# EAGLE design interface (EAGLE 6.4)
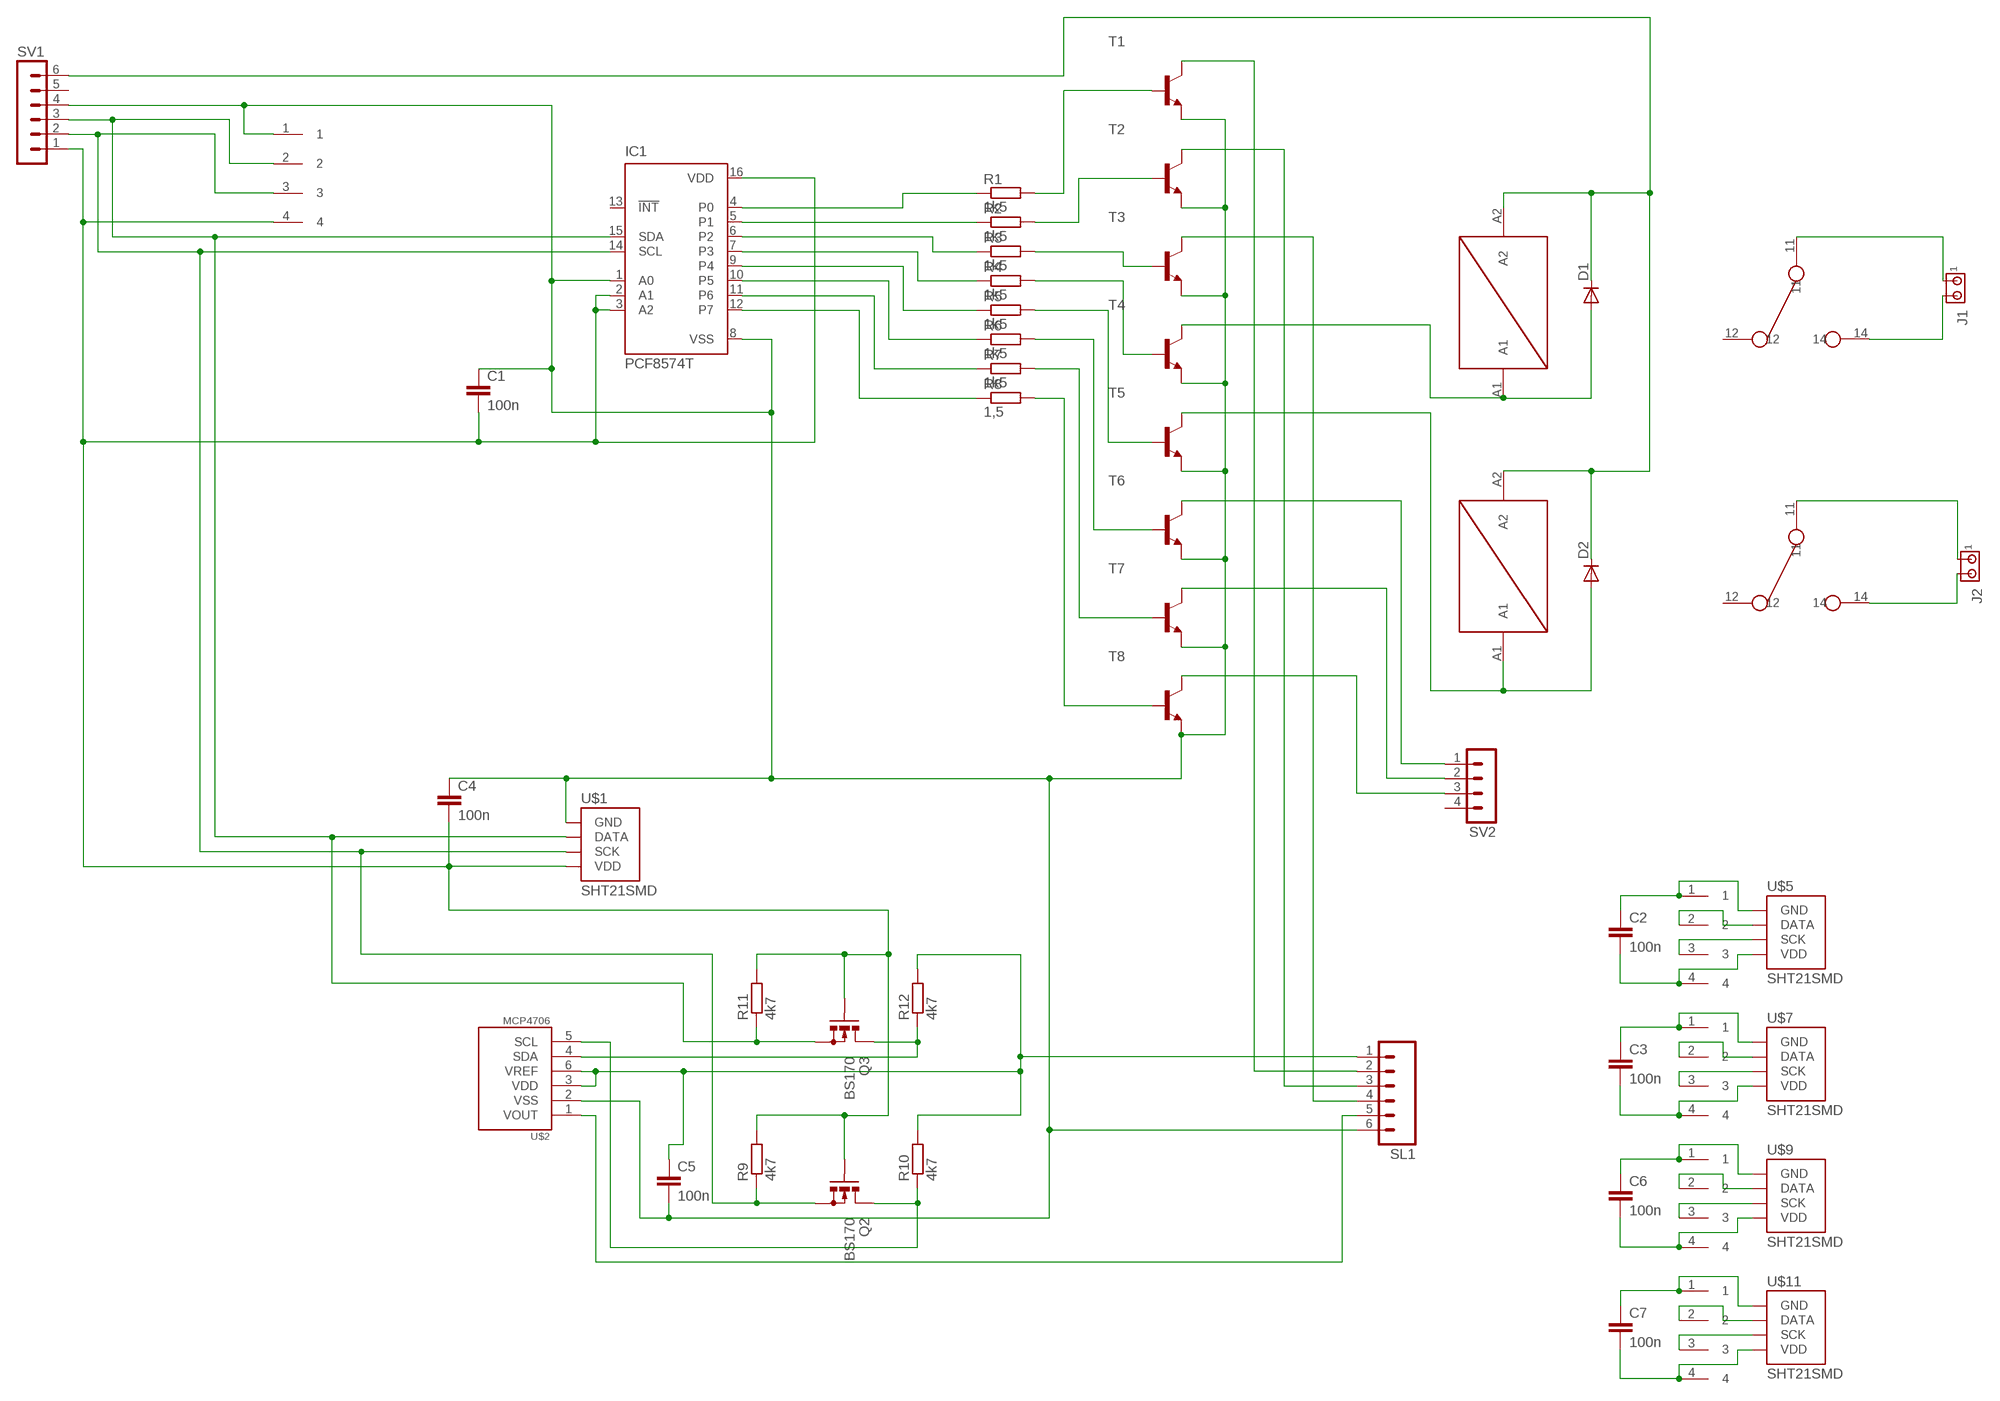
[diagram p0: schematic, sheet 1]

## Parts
C1  100n  C-EUC0805K  [C0805K]
C2  100n  C-EUC0805K  [C0805K]
C3  100n  C-EUC0805K  [C0805K]
C4  100n  C-EUC0805K  [C0805K]
C5  100n  C-EUC0805K  [C0805K]
C6  100n  C-EUC0805K  [C0805K]
C7  100n  C-EUC0805K  [C0805K]
D1  DIODE-MINIMELF  [MINIMELF]
D2  DIODE-MINIMELF  [MINIMELF]
IC1  PCF8574T  [SO16W]
J1  MTA02-156  [1X2MTA]
J2  MTA02-156  [1X2MTA]
Q2  BS170  [SOT54E]
Q3  BS170  [SOT54E]
R1  1k5  R-EU_M0805  [M0805]
R2  1k5  R-EU_M0805  [M0805]
R3  1k5  R-EU_M0805  [M0805]
R4  1k5  R-EU_M0805  [M0805]
R5  1k5  R-EU_M0805  [M0805]
R6  1k5  R-EU_M0805  [M0805]
R7  1k5  R-EU_M0805  [M0805]
R8  1,5  R-EU_M0805  [M0805]
R9  4k7  R-EU_M0805  [M0805]
R10  4k7  R-EU_M0805  [M0805]
R11  4k7  R-EU_M0805  [M0805]
R12  4k7  R-EU_M0805  [M0805]
SL1  MA06  [06PA]
SV1  MA06-1  [MA06-1]
SV2  MA04-1  [MA04-1]
T1  BCW60-NPN-SOT23-BEC  [SOT23-BEC]
T2  BCW60-NPN-SOT23-BEC  [SOT23-BEC]
T3  BCW60-NPN-SOT23-BEC  [SOT23-BEC]
T4  BCW60-NPN-SOT23-BEC  [SOT23-BEC]
T5  BCW60-NPN-SOT23-BEC  [SOT23-BEC]
T6  BCW60-NPN-SOT23-BEC  [SOT23-BEC]
T7  BCW60-NPN-SOT23-BEC  [SOT23-BEC]
T8  BCW60-NPN-SOT23-BEC  [SOT23-BEC]
U$1  SHT21SMD  [SHT21]
U$2  MCP4706  [SOT23-6]
U$3  FINDER_RELAIS  [FINDER_RELAIS]
U$4  FINDER_RELAIS  [FINDER_RELAIS]
U$5  SHT21SMD  [SHT21]
U$6  CON4PIN  [CON4PIN]
U$7  SHT21SMD  [SHT21]
U$8  CON4PIN  [CON4PIN]
U$9  SHT21SMD  [SHT21]
U$10  CON4PIN  [CON4PIN]
U$11  SHT21SMD  [SHT21]
U$12  CON4PIN  [CON4PIN]
U$13  CON4PIN  [CON4PIN]

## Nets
02: SL1.3 T2.C
03: SL1.4 T3.C
5V_ALIX: D1.C D2.C SV1.6 U$3.A2 U$4.A2
5V_LED: C5.1 R10.2 R12.2 SL1.1 U$2.3(VDD) U$2.6(VREF)
GND: C1.1 C4.1 C5.2 IC1.1(A0) IC1.8(VSS) SL1.6 SV1.4 T1.E T2.E T3.E T4.E T5.E T6.E T7.E T8.E U$1.5(GND) U$2.2(VSS) U$13.1
GND_CON: C2.1 U$5.5(GND) U$6.1
GND_CON1: C3.1 U$7.5(GND) U$8.1
GND_CON2: C6.1 U$9.5(GND) U$10.1
GND_CON3: C7.1 U$11.5(GND) U$12.1
N$1: D1.A T4.C U$3.A1
N$2: SV2.1 T6.C
N$3: IC1.4(P0) R1.1
N$4: IC1.5(P1) R2.1
N$5: IC1.6(P2) R3.1
N$6: IC1.7(P3) R4.1
N$7: D2.A T5.C U$4.A1
N$8: IC1.9(P4) R5.1
N$9: IC1.10(P5) R6.1
N$10: IC1.11(P6) R7.1
N$11: IC1.12(P7) R8.1
N$12: R1.2 T1.B
N$13: R2.2 T2.B
N$14: R3.2 T3.B
N$15: R4.2 T4.B
N$16: R5.2 T5.B
N$17: R6.2 T6.B
N$18: R7.2 T7.B
N$19: R8.2 T8.B
N$20: SV2.2 T7.C
N$21: SV2.3 T8.C
N$22: J1.1 U$3.11
N$23: Q2.D R10.1 U$2.5(SCL)
N$24: J1.2 U$3.14
N$25: J2.1 U$4.11
N$26: Q3.D R12.1 U$2.4(SDA)
N$27: J2.2 U$4.14
N$28: U$5.4(DATA) U$6.2
N$29: U$5.3(SCK) U$6.3
N$30: U$7.4(DATA) U$8.2
N$31: U$7.3(SCK) U$8.3
N$32: U$9.4(DATA) U$10.2
N$33: U$9.3(SCK) U$10.3
N$34: U$11.4(DATA) U$12.2
N$35: U$11.3(SCK) U$12.3
O1: SL1.2 T1.C
SCL: IC1.14(SCL) Q2.S R9.1 SV1.2 U$1.3(SCK) U$13.3
SDA: IC1.15(SDA) Q3.S R11.1 SV1.3 U$1.4(DATA) U$13.2
VDD: C1.2 C4.2 IC1.2(A1) IC1.3(A2) IC1.16(VDD) Q2.G Q3.G R9.2 R11.2 SV1.1 U$1.2(VDD) U$13.4
VDD_CON: C2.2 U$5.2(VDD) U$6.4
VDD_CON1: C3.2 U$7.2(VDD) U$8.4
VDD_CON2: C6.2 U$9.2(VDD) U$10.4
VDD_CON3: C7.2 U$11.2(VDD) U$12.4
VOUT: SL1.5 U$2.1(VOUT)
Unconnected: IC1.13(!INT) SV1.5 SV2.4 U$3.12 U$4.12

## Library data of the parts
C1-C7 = rcl:C-EU: CAPACITOR, European symbol
D1 D2 = diode:DIODE-: DIODE
IC1 = micro-philips:PCF8574: I2C-Bus Remote 8-bit I/O expander http://www.semiconductors.philips.com/acrobat_download/datasheets/PCF8574_4.pdf; MPN: PCF8574T/3,512; OC_FARNELL: 1201255; OC_NEWARK: 70R6870
J1 J2 = con-amp:MTA02-156: AMP connector
Q2 Q3 = transistor-small-signal:BS170: N-CHANNEL MOS FET
R1-R12 = rcl:R-EU_: RESISTOR, European symbol
SL1 = con-amp-quick:MA06: AMP QUICK CONNECTOR; OC_FARNELL: unknown; OC_NEWARK: unknown
SV1 = con-lstb:MA06-1: PIN HEADER; OC_FARNELL: unknown; OC_NEWARK: unknown
SV2 = con-lstb:MA04-1: PIN HEADER; OC_FARNELL: unknown; OC_NEWARK: unknown
T1-T8 = transistor:*-NPN-: NPN Transistror BF959 corrected 2008.03.06
U$1 U$5 U$7 U$9 U$11 = parts:SHT21: SHT21/25 Humdity Sensor Sensirion humdity sensor.
U$2 = parts:MCP4706: MCP4706 I2C DAC
U$3 U$4 = parts:FINDER_RELAIS: Finder Relais 36.11-4001
U$6 U$8 U$10 U$12 U$13 = parts:CON4PIN

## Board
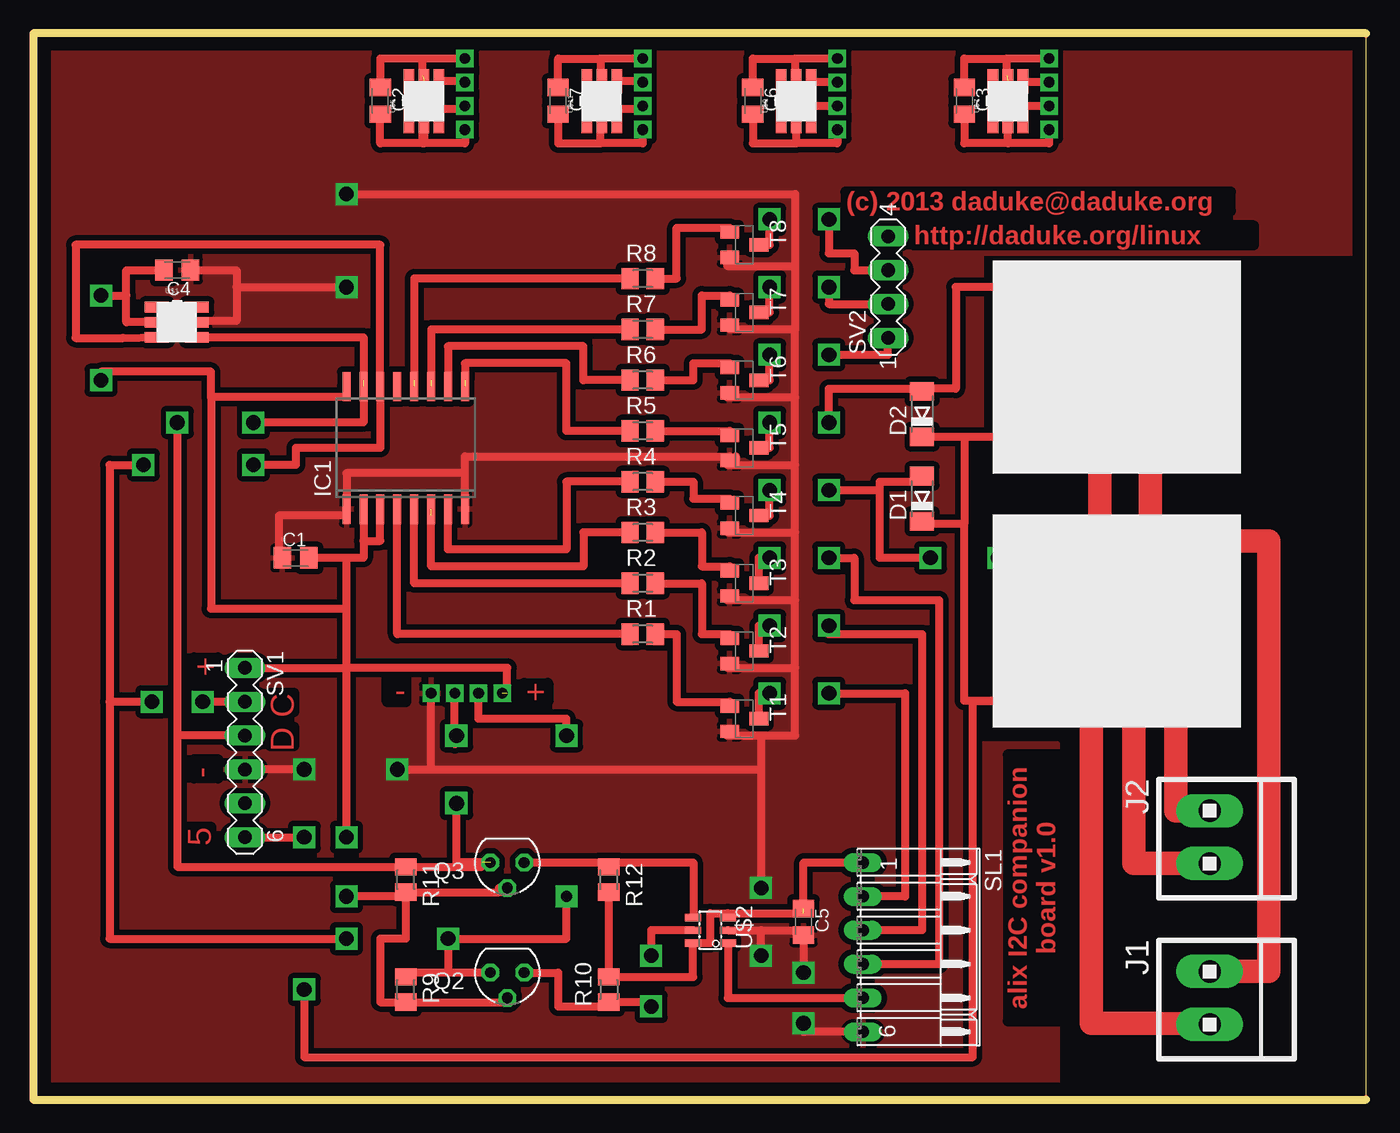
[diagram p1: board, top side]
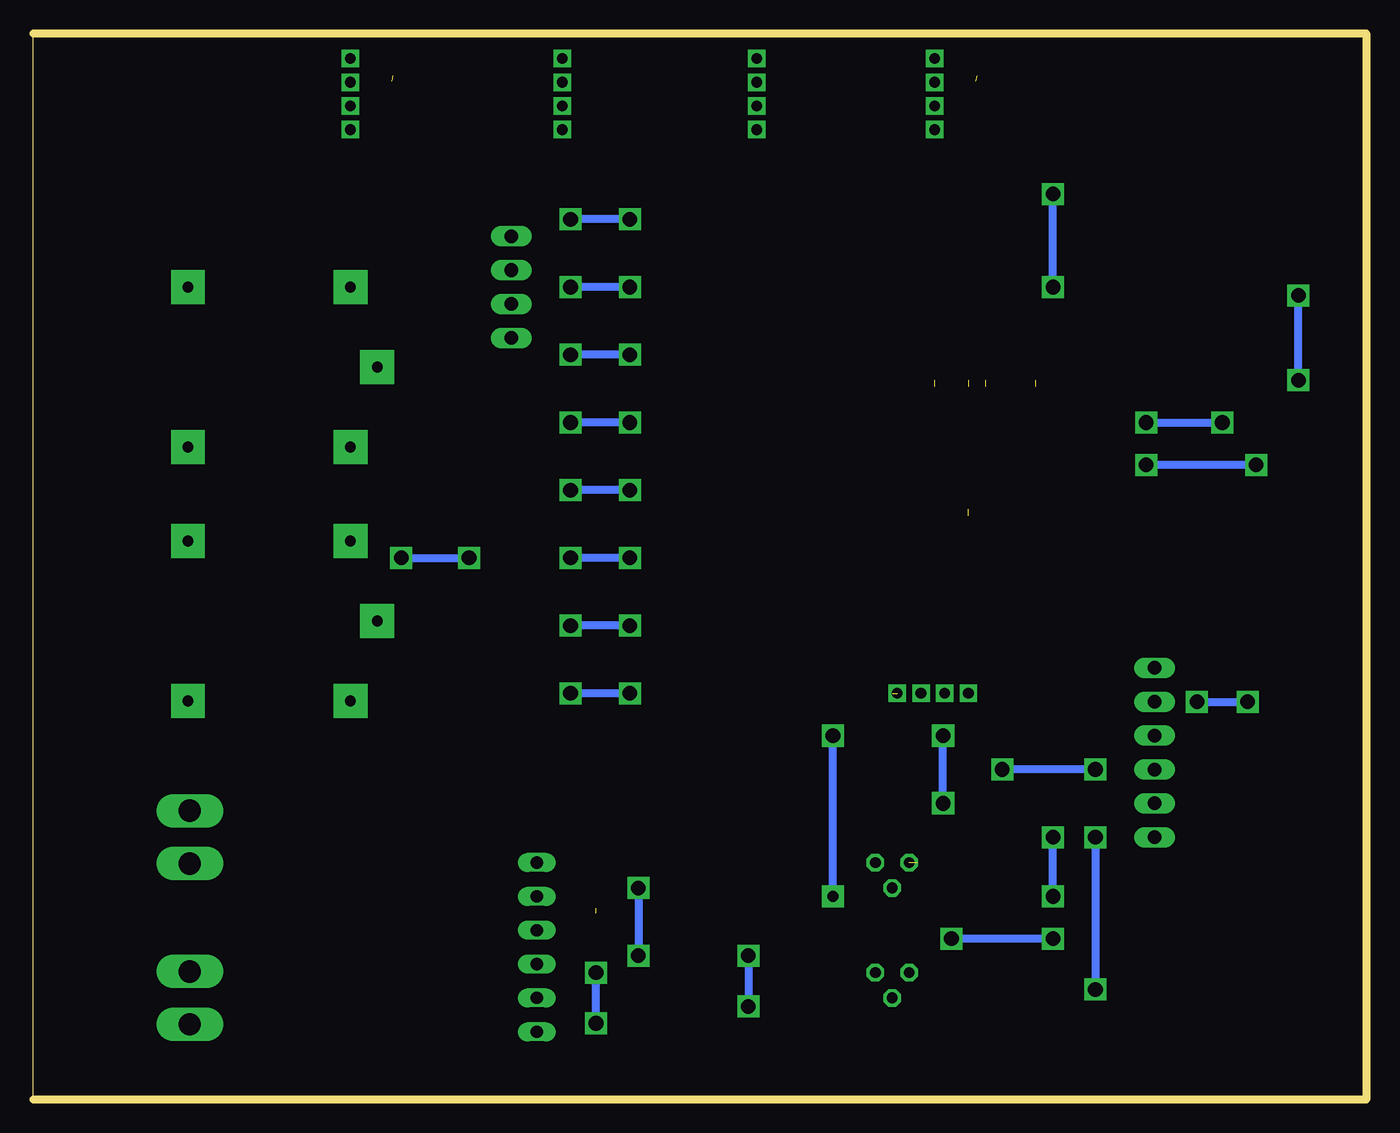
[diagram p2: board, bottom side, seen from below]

Size 100 x 80 mm. Coordinates in mm from the lower left corner, seen from the top.
Outline: 0,0 100,0 100,80 0,80 0,0
Copper layers (1*16): Top 0.035mm / dielectric 1.5mm / Bottom 0.035mm
Design rules "default": minimum track width 10mil, minimum drill 24mil, track to track 8mil, track to pad 8mil, pad to pad 8mil, via to via 8mil, smd to smd 8mil, copper to edge 40mil, drill to drill 8mil, minimum pad ring 10mil, minimum via ring 8mil, stop-mask expansion 4mil, vias tented up to drill 0mil, thermal gap 10mil

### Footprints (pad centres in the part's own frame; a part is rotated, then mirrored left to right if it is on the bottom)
C0805K = smd 1.3 x 1.6: 1 -1,0; 2 1,0
MINIMELF = smd 1.4 x 1.8: A 1.7,0; C -1.7,0
SO16W = smd 0.6 x 2.2: 1 -4.445,-4.6; 2 -3.175,-4.6; 3 -1.905,-4.6; 4 -0.635,-4.6; 5 0.635,-4.6; 6 1.905,-4.6; 7 3.175,-4.6; 8 4.445,-4.6; 9 4.445,4.6; 10 3.175,4.6; 11 1.905,4.6; 12 0.635,4.6; 13 -0.635,4.6; 14 -1.905,4.6; 15 -3.175,4.6; 16 -4.445,4.6
1X2MTA = drill 1.676 long: 1 1.981,0; 2 -1.981,0
SOT54E = drill 0.813 octagon: D -1.27,0; G 0,1.905; S 1.27,0
M0805 = smd 1.3 x 1.6: 1 -0.95,0; 2 0.95,0
06PA = drill 0.914 long: 1 -6.35,0; 2 -3.81,0; 3 -1.27,0; 4 1.27,0; 5 3.81,0; 6 6.35,0
MA06-1 = drill 1.016 long: 1 -6.35,0; 2 -3.81,0; 3 -1.27,0; 4 1.27,0; 5 3.81,0; 6 6.35,0
MA04-1 = drill 1.016 long: 1 -3.81,0; 2 -1.27,0; 3 1.27,0; 4 3.81,0
SOT23-BEC = smd 1 x 1.4: B -0.95,-1.1; C 0,1.1; E 0.95,-1.1
SHT21 = smd 1.8 x 0.8: 1 -2.16,1.667; 2 -2.16,0.54; 3 -2.16,-0.587; 4 0.84,-0.587; 5 0.84,0.54; 6 0.84,1.667
SOT23-6 = smd 0.55 x 1.2: 1 -0.95,-1.3; 2 0,-1.3; 3 0.95,-1.3; 4 0.95,1.3; 5 0,1.3; 6 -0.95,1.3
FINDER_RELAIS = drill 0.8 pad 2.54 square: 11 -2,-6; 12 12.2,-12; 14 12.2,0; A1 0,0; A2 0,-12
CON4PIN = drill 0.8 square: 1 0,0; 2 1.778,0; 3 3.556,0; 4 5.334,0

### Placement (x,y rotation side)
C1  19.68,40.64 0 top
C2  26.04,74.93 270 top
C3  69.85,74.93 270 top
C4  10.79,62.23 180 top
C5  57.78,13.34 270 top
C6  53.98,74.93 270 top
C7  39.37,74.93 270 top
D1  66.67,45.09 90 top
D2  66.67,51.44 90 top
IC1  27.94,48.9 0 top
J1  88.27,7.62 270 top
J2  88.27,19.68 270 top
Q2  35.56,9.53 180 top
Q3  35.56,17.78 180 top
R1  45.72,34.92 0 top
R2  45.72,38.73 0 top
R3  45.72,42.55 0 top
R4  45.72,46.35 0 top
R5  45.72,50.16 0 top
R6  45.72,53.98 0 top
R7  45.72,57.78 0 top
R8  45.72,61.59 0 top
R9  27.94,8.26 270 top
R10  43.18,8.26 90 top
R11  27.94,16.51 270 top
R12  43.18,16.51 270 top
SL1  62.23,11.43 270 top
SV1  15.88,26.04 270 top
SV2  64.14,60.96 90 top
T1  53.34,28.57 270 top
T2  53.34,33.66 270 top
T3  53.34,38.73 270 top
T4  53.34,43.81 270 top
T5  53.34,48.9 270 top
T6  53.34,53.98 270 top
T7  53.34,59.05 270 top
T8  53.34,64.14 270 top
U$1  11.43,57.78 0 top
U$2  50.8,12.7 90 top
U$3  76.2,41.91 0 top
U$4  76.2,60.96 0 top
U$5  29.84,75.56 90 top
U$6  32.38,78.11 270 top
U$7  73.66,75.56 90 top
U$8  76.2,78.11 270 top
U$9  57.78,75.56 90 top
U$10  60.33,78.11 270 top
U$11  43.18,75.56 90 top
U$12  45.72,78.11 270 top
U$13  29.84,30.48 0 top

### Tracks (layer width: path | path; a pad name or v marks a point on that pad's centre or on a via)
02  (via drill 1.1)
  Top 0.61: T2.C 54.44,35.56 v55.24,35.56 | v59.69,35.56 59.69,34.92 66.67,34.92 66.67,12.7 SL1.3
  Bottom 0.61: v55.24,35.56 v59.69,35.56
03  (via drill 1.1)
  Top 0.61: T3.C 54.44,40.64 v55.24,40.64 | SL1.4 67.94,10.16 67.94,37.47 61.59,37.47 61.59,40.64 v59.69,40.64
  Bottom 0.61: v55.24,40.64 v59.69,40.64
5V_ALIX  (via drill 1.1 pad 0.3)
  Top 0.61: SV1.6 v20.32,19.68 | v20.32,8.26 20.32,3.17 70.48,3.17 70.48,29.91 U$3.A2 69.85,29.91 69.85,43.18 | 69.85,43.18 66.67,43.18 D1.C | D2.C 69.85,49.73 | 69.85,49.73 69.85,43.18 | 69.85,49.73 76.2,49.73 U$4.A2
  Bottom 0.61: v20.32,19.68 v20.32,8.26
5V_LED  (1 unrouted)
  Top 0.61: R12.2 R10.2 49.5,9.21 U$2.6 50.8,11.75 50.8,13.97 52.1,13.97 | U$2.3 52.1,13.97 | 52.1,13.97 57.78,13.97 57.78,17.78 SL1.1
GND  (via drill 1.1)
  Top 0.61: T8.E 52.07,62.87 52.07,62.55 57.15,62.55 | 57.15,62.55 57.15,57.78 | 57.15,57.78 52.24,57.78 T7.E | T6.E 52.07,53.02 52.07,52.7 57.15,52.7 | 57.15,52.7 57.15,57.78 | T5.E 52.07,47.95 52.07,47.62 57.15,47.62 | 57.15,47.62 57.15,52.7 | T4.E 52.07,42.87 52.07,42.55 57.15,42.55 | 57.15,42.55 57.15,47.62 | T3.E 52.07,37.78 52.07,37.47 57.15,37.47 | 57.15,37.47 57.15,42.55 | T2.E 52.07,32.7 52.07,32.38 57.15,32.38 | 57.15,32.38 57.15,37.47 | T1.E 52.07,27.62 52.07,27.3 54.61,27.3 | 54.61,27.3 57.15,27.3 57.15,32.38 | U$2.2 54.61,12.7 | v54.61,10.79 54.61,12.7 | 54.61,12.7 57.78,12.7 C5.2 v57.78,9.53 | SL1.6 57.78,5.08 v57.78,5.71 | 54.61,27.3 54.61,24.77 | 54.61,24.77 v54.61,15.88 | IC1.8 32.38,46.99 | 32.38,46.99 23.5,46.99 IC1.1 23.5,43.81 18.41,43.81 18.41,40.64 C1.1 | 32.38,46.99 32.38,48.26 52.24,48.26 T5.E | 52.7,48.26 52.7,47.95 T5.E | 54.61,24.77 v27.3,24.77 29.84,24.77 U$13.1 | v20.32,24.77 SV1.4 | 15.24,60.96 v23.5,60.96 | v23.5,67.94 57.15,67.94 57.15,62.55 | C4.1 15.24,62.23 15.24,58.42 12.27,58.42 U$1.5
  Bottom 0.61: v57.78,5.71 v57.78,9.53 | v54.61,15.88 v54.61,10.79 | v20.32,24.77 v27.3,24.77 | v23.5,60.96 v23.5,67.94
  pour Top (isolate 0.406): 0.64,79.38 99.69,79.38 99.69,63.5 71.12,63.5 71.12,26.67 76.83,26.67 76.83,0.64 0.64,0.64
GND_CON  (1 unrouted)
  Top 0.61: U$6.1 29.21,78.11 | 29.21,76.83 29.21,78.11 | 29.21,78.11 26.04,78.11 C2.1
GND_CON1  (1 unrouted)
  Top 0.61: U$8.1 73.03,78.11 | 73.03,76.83 73.03,78.11 | C3.1 69.85,78.11 73.03,78.11
GND_CON2
  Top 0.61: U$10.1 57.15,78.11 | 57.15,78.11 57.15,76.41 U$9.5 | C6.1 53.98,78.11 57.15,78.11
GND_CON3
  Top 0.61: U$12.1 42.55,78.11 | 42.55,78.11 42.55,76.41 U$11.5 | C7.1 39.37,78.11 42.55,78.11
N$1  (via drill 1.1, 1.1 pad 0.3)
  Top 0.61: T4.C 55.24,43.81 v55.24,45.72 | v59.69,45.72 63.5,45.72 | 63.5,45.72 63.5,46.35 66.67,46.35 D1.A | v67.31,40.64 63.5,40.64 63.5,45.72 | U$3.A1 72.39,41.91 v72.39,40.64
  Bottom 0.61: v55.24,45.72 v59.69,45.72 | v72.39,40.64 v67.31,40.64
N$2  (via drill 1.1)
  Top 0.61: T6.C 55.24,53.98 v55.24,55.88 | v59.69,55.88 64.14,55.88 SV2.1
  Bottom 0.61: v55.24,55.88 v59.69,55.88
N$3
  Top 0.61: R1.1 27.3,34.92 IC1.4
N$4
  Top 0.61: R2.1 28.57,38.73 IC1.5
N$5  (1 unrouted)
  Top 0.61: R3.1 41.27,42.55 41.27,40.01 29.84,40.01 29.84,43.81
N$6
  Top 0.61: R4.1 40.01,46.35 40.01,41.27 31.11,41.27 IC1.7
N$7  (via drill 1.1)
  Top 0.61: T5.C 55.24,48.9 v55.24,50.8 | v59.69,50.8 59.69,53.34 66.67,53.34 | U$4.A1 69.22,60.96 69.22,53.34 66.67,53.34 | 66.67,53.34 D2.A
  Bottom 0.61: v55.24,50.8 v59.69,50.8
N$8  (1 unrouted)
  Top 0.61: R5.1 40.01,50.16 40.01,55.24 32.38,55.24 32.38,53.98
N$9
  Top 0.61: R6.1 41.27,53.98 41.27,56.52 31.11,56.52 IC1.10
N$10  (1 unrouted)
  Top 0.61: R7.1 29.84,57.78 29.84,53.98
N$11  (1 unrouted)
  Top 0.61: R8.1 28.57,61.59 28.57,53.98
N$12
  Top 0.61: R1.2 48.26,34.92 48.26,29.84 52.24,29.84 T1.B
N$13
  Top 0.61: R2.2 50.16,38.73 50.16,34.92 52.24,34.92 T2.B
N$14
  Top 0.61: R3.2 50.16,42.55 50.16,40.01 52.24,40.01 T3.B
N$15
  Top 0.61: R4.2 49.53,46.35 49.53,45.09 52.24,45.09 T4.B
N$16
  Top 0.61: R5.2 52.24,50.16 T5.B
N$17
  Top 0.61: R6.2 49.53,53.98 49.53,55.24 52.24,55.24 T6.B
N$18
  Top 0.61: R7.2 50.16,57.78 50.16,60.33 52.24,60.33 T7.B
N$19
  Top 0.61: R8.2 48.26,61.59 48.26,65.41 52.24,65.41 T8.B
N$20  (via drill 1.1)
  Top 0.61: T7.C 55.24,59.05 v55.24,60.96 | v59.69,60.96 59.69,59.69 SV2.2
  Bottom 0.61: v55.24,60.96 v59.69,60.96
N$21  (via drill 1.1)
  Top 0.61: T8.C 55.24,64.14 v55.24,66.04 | v59.69,66.04 59.69,63.5 61.59,63.5 61.59,62.23 SV2.3
  Bottom 0.61: v55.24,66.04 v59.69,66.04
N$22
  Top 1.778: U$3.11 79.38,35.91 79.38,5.71 84.45,5.71 J1.1
N$23  (via drill 1.1)
  Top 0.61: Q2.D 39.37,9.53 39.37,6.99 43.18,6.99 R10.1 46.35,7.3 v46.35,6.99 | U$2.5 46.35,12.7 v46.35,10.79
  Bottom 0.61: v46.35,10.79 v46.35,6.99
N$24
  Top 1.778: J1.2 92.71,9.6 92.71,41.91 U$3.14
N$25
  Top 1.27: 74.2,55.24 U$4.11
  Top 1.778: J2.1 82.55,17.7 82.55,38.73 80.01,38.73 80.01,55.24 74.2,55.24
N$26
  Top 0.61: Q3.D 43.18,17.78 | R12.1 43.18,17.78 | 43.18,17.78 49.53,17.78 49.53,13.65 U$2.4
N$27
  Top 1.778: J2.2 85.72,21.67 85.72,39.37 83.82,41.91 83.82,60.96 U$4.14
N$28
  Top 0.61: U$6.2 32.38,76.41 U$5.4
N$29
  Top 0.61: U$6.3 32.38,74.3 30.48,74.3 30.48,73.41 U$5.3
N$30
  Top 0.61: U$8.2 74.25,76.33 U$7.4
N$31
  Top 0.61: U$8.3 74.25,74.55 U$7.3
N$32
  Top 0.61: U$10.2 58.37,76.33 U$9.4
N$33
  Top 0.61: U$10.3 58.37,74.55 U$9.3
N$34
  Top 0.61: U$12.2 45.72,76.41 U$11.4
N$35
  Top 0.61: U$12.3 45.72,74.3 43.81,74.3 43.81,73.41 U$11.3
O1  (via drill 1.1)
  Top 0.61: T1.C 54.44,30.48 v55.24,30.48 | v59.69,30.48 65.41,30.48 65.41,15.24 SL1.2
  Bottom 0.61: v55.24,30.48 v59.69,30.48
SCL  (via drill 0.8 pad 1.68, 1.1, 1.1 pad 1.68)
  Top 0.61: Q2.S 31.11,9.53 | 31.11,9.53 27.94,9.53 R9.1 | v16.51,47.62 19.68,47.62 19.68,48.9 26.04,48.9 IC1.14 26.04,64.14 3.17,64.14 3.17,57.15 6.73,57.15 U$1.3 | 5.71,29.84 5.71,47.62 v8.26,47.62 | 5.71,29.84 5.71,12.06 v23.5,12.06 | 31.11,9.53 v31.11,12.06 40.01,12.06 v40.01,15.24 | v8.89,29.84 5.71,29.84 | SV1.2 v12.7,29.84 | v40.01,27.3 40.01,28.57 33.4,28.57 U$13.3
  Bottom 0.61: v23.5,12.06 v31.11,12.06 | v8.26,47.62 v16.51,47.62 | v12.7,29.84 v8.89,29.84 | v40.01,15.24 v40.01,27.3
SDA  (via drill 1.1, 1.1 pad 1.68)  (2 unrouted)
  Top 0.61: IC1.15 24.77,50.8 v16.51,50.8 | v10.79,50.8 10.79,27.3 | 10.79,27.3 10.79,17.46 R11.1 33.66,17.46 33.66,17.78 31.75,17.78 v31.75,22.23 | SV1.3 10.79,27.3 | U$1.4 24.77,57.2 24.77,53.98 | v31.75,27.3 31.62,26.67 U$13.2
  Bottom 0.61: v16.51,50.8 v10.79,50.8 | v31.75,22.23 v31.75,27.3
VDD  (via drill 1.1)  (1 unrouted)
  Top 0.61: R11.2 34.92,15.56 | 34.92,15.56 34.92,15.88 | Q2.G 35.56,7.3 R9.2 26.04,7.3 26.04,12.06 27.94,12.06 R11.2 | IC1.3 26.04,41.91 24.77,41.91 IC1.2 24.77,40.64 23.5,40.64 | 23.5,40.64 C1.2 | IC1.16 23.5,52.7 13.34,52.7 | Q3.G 35.56,15.56 34.92,15.56 | R11.2 27.94,15.24 v23.5,15.24 | 13.34,52.7 13.34,36.83 23.5,36.83 | v23.5,19.68 23.5,32.38 | 23.5,32.38 23.5,36.83 | SV1.1 23.5,32.38 | 23.5,36.83 23.5,40.64 | U$1.2 6.99,58.33 6.99,60.33 | 6.99,60.33 6.99,62.23 C4.2 | 13.34,52.7 13.34,54.61 5.08,54.61 v5.08,53.98 | v5.08,60.33 6.99,60.33 | 35.56,30.48 35.56,32.38 23.5,32.38
  Bottom 0.61: v23.5,15.24 v23.5,19.68 | v5.08,53.98 v5.08,60.33
VDD_CON
  Top 0.61: 29.21,71.75 29.21,73.41 U$5.2 29.3,71.75 | 29.3,71.75 26.04,71.75 C2.2 | U$6.4 32.38,71.75 29.3,71.75
VDD_CON1
  Top 0.61: U$8.4 76.2,71.75 73.12,71.75 | 73.12,71.75 U$7.2 | C3.2 69.85,71.75 73.12,71.75
VDD_CON2
  Top 0.61: U$10.4 60.33,71.75 57.24,71.75 | 57.24,71.75 U$9.2 | C6.2 53.98,71.75 57.24,71.75
VDD_CON3
  Top 0.61: U$12.4 45.72,71.75 42.55,71.75 | 42.55,71.75 42.55,73.41 U$11.2 | C7.2 39.37,71.75 42.55,71.75
VOUT
  Top 0.61: U$2.1 52.1,7.62 SL1.5

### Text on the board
Top: (c) 2013 daduke@daduke.org | http://daduke.org/linux | + | C | - | + | D | - | 5 | alix I2C companion / board v1.0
